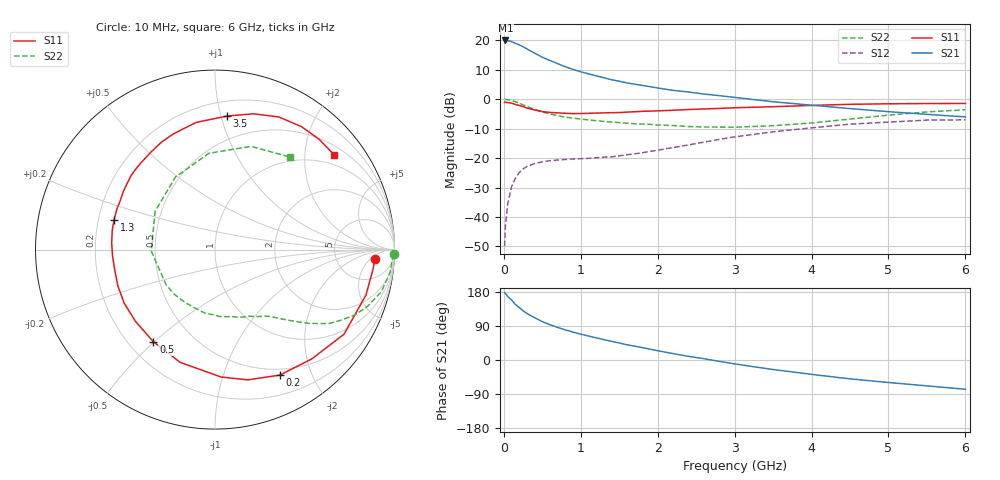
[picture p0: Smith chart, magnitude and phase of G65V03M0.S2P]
! SIEMENS Small Signal Semiconductors
! BFG193
! Si NPN RF Bipolar Junction Transistor in SOT223
! VCE = 5 V  IC = 3 mA
! Common Emitter S-Parameters:  August  1996
# GHz  S  MA  R  50
!  f  S11  S21  S12  S22
! GHz  MAG  ANG  MAG  ANG  MAG  ANG  MAG  ANG
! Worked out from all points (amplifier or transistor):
!   36 points, 10 MHz to 6 GHz, reference 50 ohm
!   highest |S21| = 20.0 dB at 20 MHz (marker M1)
!   |S21| within 3 dB of that: start of sweep to 308.9 MHz
!   unconditionally stable (mu >= 1): 1.285 GHz to 2.501 GHz
!   at 250 MHz: K = 0.23, MSG = 20.7 dB, |S12| = -23.7 dB
!   at 1.4 GHz: K = 1.07, MAG = 11.5 dB, |S12| = -19.6 dB
!   at 6 GHz: K = 0.91, MSG = 0.5 dB, |S12| = -7.0 dB
!   S11 on the Smith chart (normalised r, x): 10 MHz: 14, -7; 200 MHz: 0.42, -1.56; 500 MHz: 0.30, -0.50; 1.3 GHz: 0.27, +0.13; 3.5 GHz: 0.31, +1.04; 6 GHz: 0.72, +2.70
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0.01  0.8927 -3.3  9.959 177.5  0.0032 92.9  0.995 -1.5
0.02  0.8873 -7.0  9.962 176.1  0.0069 85.2  0.9896 -2.9
0.05  0.8784 -16.7  9.844 167.8  0.0166 80.9  0.9837 -7.4
0.1  0.8597 -33.2  9.525 158.2  0.0325 72.8  0.9563 -14.2
0.15  0.8135 -48.5  8.914 146.8  0.0457 63.9  0.9067 -20.4
0.2  0.7868 -62.7  8.368 138.5  0.0567 58.1  0.8582 -25.2
0.25  0.7486 -75.8  7.783 129.9  0.0655 52.1  0.8017 -29.5
0.3  0.7106 -87.3  7.157 122.9  0.0721 47.7  0.7564 -33.0
0.4  0.6577 -107.1  6.064 111.6  0.0808 40.2  0.6701 -37.9
0.5  0.6179 -123.7  5.17 101.2  0.0867 35.0  0.6081 -41.3
0.6  0.5965 -137.9  4.546 93.1  0.0906 32.1  0.5628 -44.2
0.7  0.5876 -149.5  4.018 85.9  0.0929 30.0  0.5268 -46.8
0.9  0.5701 -168.4  3.214 73.6  0.097 28.0  0.4771 -51.1
1.1  0.5769 176.3  2.696 63.3  0.0994 28.3  0.4455 -56.8
1.3  0.5863 163.5  2.32 53.9  0.1039 29.9  0.4192 -62.3
1.6  0.6049 147.6  1.894 40.2  0.1141 32.3  0.3928 -73.1
2.2  0.6502 123.2  1.415 16.9  0.1513 34.3  0.3581 -98.8
2.8  0.6981 103.8  1.15 -3.6  0.2082 29.0  0.3367 -132.2
3.5  0.7469 84.9  0.907 -25.2  0.2798 14.9  0.3554 -178.8
4.5  0.8202 64.3  0.694 -49.8  0.3777 -7.6  0.4605 118.6
5.5  0.8451 46.7  0.554 -68.3  0.4425 -35.5  0.6092 70.8
6  0.8486 38.4  0.502 -77.2  0.4474 -50.9  0.6636 51.0
